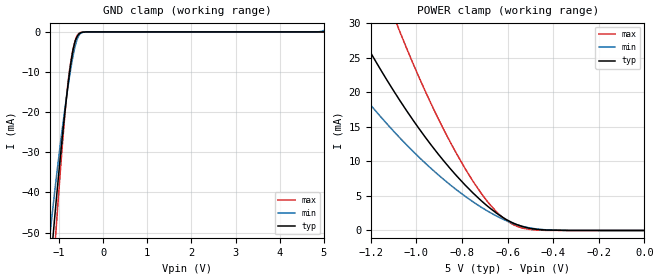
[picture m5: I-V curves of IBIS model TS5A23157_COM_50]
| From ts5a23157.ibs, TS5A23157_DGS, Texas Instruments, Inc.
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[Model]   TS5A23157_COM_50
Model_type  Terminator
| variable   typ   min   max
C_comp   15.50pF   11.56pF   16.98pF
| C_tri-state   15.50pF   11.56pF   16.98pF
[Temperature Range]   40   100   -40
| Ambient temperature   25   85   -40
[Voltage range]   5   4.5   5.5
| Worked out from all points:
|   GND clamp passes 1 mA (typ) near -0.58 V on its own axis
|   POWER clamp passes 1 mA (typ) near -0.57 V on its own axis
[GND Clamp]
| TS5A23157_COM_50
|   Voltage   I(typ)   I(min)   I(max)
-5V       -677.8mA   -564.8mA   -796.7mA
-1.235V   -63.47mA   -53.4mA    -76.12mA
-1.19V    -57.63mA   -48.81mA   -68.67mA
-1.145V   -51.9mA    -44.31mA   -61.35mA
-1.105V   -46.92mA   -40.4mA    -54.96mA
-1.085V   -44.47mA   -38.47mA   -51.81mA
-1.065V   -42.04mA   -36.56mA   -48.69mA
-900mV    -23.3mA    -21.75mA   -24.66mA
-785mV    -12.04mA   -12.66mA   -11.4mA
-665mV    -3.569mA   -4.972mA   -3.368mA
-530mV    -354uA     -556.9uA   -200.8uA
5V        5.344nA    343.5uA    5.11nA
[POWER Clamp]
| TS5A23157_COM_50
|   Voltage   I(typ)   I(min)   I(max)
-5V       455.3mA    346.4mA    640.4mA
-1.47V    42.81mA    29.97mA    67.24mA
-1.435V   40.4mA     28.29mA    63.42mA
-1.25V    28.55mA    20.1mA     44.51mA
-1.1V     20.18mA    14.34mA    30.99mA
-1.07V    18.64mA    13.28mA    28.5mA
-935mV    12.33mA    8.937mA    18.25mA
-785mV    6.514mA    4.906mA    8.864mA
-695mV    3.703mA    2.939mA    4.451mA
-620mV    1.864mA    1.626mA    1.83mA
-505mV    326.4uA    374.1uA    158.4uA
-84.45fV  5.344nA    5.865nA    5.638nA
